| TEXAS INSTRUMENTS INCORPORATED
| Standard Linear and Logic Group
| IBIS Model of SN74AUCH16374
| 16-Bit Edge-Triggered D-Type Flip-Flop with 3-State Outputs
| This file contains package information for the following:
|  TSSOP 48-pin (DGG) package as [Component] AUCH16374_DGG
|  TVSOP 48-pin (DGV) package as [Component] AUCH16374_DGV
| This device can be powered at the following Vccs:
|  2.5 volt Vcc
|  1.8 volt Vcc
|  1.5 volt Vcc
|  1.2 volt Vcc
|  0.8 volt Vcc
| This file provides unique models under the [Model Selector] for each Vcc.
| For operation at a specific Vcc, select the appropriate model after each
| [Model Selector] keyword.
[IBIS Ver]   3.2
[Comment char]  |_char
[File Name]   sn74auch16374.ibs
[File Rev]   1.1 | x_die
[Date]   June 26, 2003
[Source]   Data created from TI-SPICE simulations at TI-SLL.
[Notes]   The following is an IBIS list for the AUCH16374.
   Please contact sllibis@ti.com with questions and
   comments concerning SLL IBIS models.
   -End point warning due to AC and DC mismatch.
   -Non-monotonic data in ground-clamp due to bus-hold
   -The waveforms for the AUCH16374_OUT Power Clamp ,Pullup,
   and Pulldown are caused by the circuitry that helps reduce
   overshoot and undershoot in transmission lines (EMI).
   These waveforms are norimal for this particular design.
   -Power clamp data deleted as there is no power-clamp diode.
[Disclaimer] Property of Texas Instruments Incorporated.  Unauthorized
   reproduction and/or distribution is strictly prohibited.
   This product is protected under copyright law.
   Created  2003, (C) Copyright  2003, Texas Instruments
   Incorporated, All Rights Reserved
   UNLESS THERE IS A SIGNED, WRITTEN AGREEMENT TO THE
   CONTRARY, TEXAS INSTRUMENTS (TI) IS PROVIDING THE IBIS
   MODELS  AND WITHOUT ANY WARRANTY, EXPRESSED OR
   IMPLIED.  TI assumes no liability for:
   1) the accuracy of the IBIS models provided to your
   company;
   2) the proper functioning of these IBIS Models in your
   design or for any resulting applications; or
   3) infringement of patents, copyrights or intellectual
   property rights resulting from your use of these IBIS
   models.
   TI provides IBIS Models as a service to our customers.
   You and your company shall not distribute, sell or give
   these models to anyone else without prior written
   permission from TI.
   TI reserves the right to make changes to our products or
   to discontinue any semiconductor product or service
   without notice, and advises our customers to obtain the
   latest version of relevant information to verify, before
   placing orders, that the information being relied on is
   current.
   Please be aware that your receipt and use of the IBIS
   information provided shall serve as acceptance of these
   terms and conditions.  If you do not accept these terms,
   you should return or destroy the IBIS models and any
   other accompanying information immediately.
| Component AUCH16374_DGG 48-pin TSSOP
[Component]   AUCH16374_DGG
[Manufacturer]   Texas Instruments, Inc.
[Package]
|   typ   min   max
R_pkg   6.200e-02   5.000e-02   7.800e-02
L_pkg   3.527e-09   3.128e-09   4.255e-09
C_pkg   5.300e-13   4.170e-13   6.850e-13
[Pin]   signal_name   model_name   R_pin   L_pin   C_pin
1   1NOE   AUCH16374_OEIN   5.000e-02   4.250e-09   6.710e-13
2   1Q1   AUCH16374_OUT   5.700e-02   3.956e-09   6.740e-13
3   1Q2   AUCH16374_OUT   7.100e-02   3.922e-09   6.190e-13
4   GND   GND   7.800e-02   3.841e-09   6.180e-13
5   1Q3   AUCH16374_OUT   5.600e-02   3.535e-09   5.550e-13
6   1Q4   AUCH16374_OUT   5.800e-02   3.464e-09   5.030e-13
7   VCC   POWER   6.000e-02   3.362e-09   4.980e-13
8   1Q5   AUCH16374_OUT   6.100e-02   3.293e-09   4.620e-13
9   1Q6   AUCH16374_OUT   6.300e-02   3.240e-09   4.550e-13
10   GND   GND   6.300e-02   3.175e-09   4.420e-13
11   1Q7   AUCH16374_OUT   6.400e-02   3.153e-09   4.290e-13
12   1Q8   AUCH16374_OUT   6.500e-02   3.128e-09   4.180e-13
13   2Q1   AUCH16374_OUT   6.500e-02   3.128e-09   4.180e-13
14   2Q2   AUCH16374_OUT   6.400e-02   3.154e-09   4.290e-13
15   GND   GND   6.300e-02   3.174e-09   4.420e-13
16   2Q3   AUCH16374_OUT   6.300e-02   3.241e-09   4.550e-13
17   2Q4   AUCH16374_OUT   6.100e-02   3.293e-09   4.620e-13
18   VCC   POWER   6.000e-02   3.362e-09   4.970e-13
19   2Q5   AUCH16374_OUT   5.800e-02   3.464e-09   5.030e-13
20   2Q6   AUCH16374_OUT   5.600e-02   3.537e-09   5.600e-13
21   GND   GND   7.700e-02   3.839e-09   6.260e-13
22   2Q7   AUCH16374_OUT   7.100e-02   3.917e-09   6.270e-13
23   2Q8   AUCH16374_OUT   5.800e-02   3.955e-09   6.850e-13
24   2NOE   AUCH16374_OEIN   5.200e-02   4.255e-09   6.790e-13
25   2CLK   AUCH16374_CLKIN   5.100e-02   4.254e-09   6.760e-13
26   2D8   AUCH16374_IN   5.800e-02   3.957e-09   6.790e-13
27   2D7   AUCH16374_IN   7.100e-02   3.920e-09   6.210e-13
28   GND   GND   7.800e-02   3.843e-09   6.220e-13
29   2D6   AUCH16374_IN   5.600e-02   3.539e-09   5.600e-13
30   2D5   AUCH16374_IN   5.800e-02   3.466e-09   5.030e-13
31   VCC   POWER   6.000e-02   3.363e-09   4.970e-13
32   2D4   AUCH16374_IN   6.100e-02   3.294e-09   4.620e-13
33   2D3   AUCH16374_IN   6.300e-02   3.241e-09   4.540e-13
34   GND   GND   6.300e-02   3.175e-09   4.410e-13
35   2D2   AUCH16374_IN   6.400e-02   3.153e-09   4.290e-13
36   2D1   AUCH16374_IN   6.500e-02   3.129e-09   4.170e-13
37   1D8   AUCH16374_IN   6.500e-02   3.129e-09   4.170e-13
38   1D7   AUCH16374_IN   6.400e-02   3.152e-09   4.290e-13
39   GND   GND   6.400e-02   3.176e-09   4.410e-13
40   1D6   AUCH16374_IN   6.300e-02   3.241e-09   4.540e-13
41   1D5   AUCH16374_IN   6.100e-02   3.293e-09   4.620e-13
42   VCC   POWER   6.000e-02   3.363e-09   4.970e-13
43   1D4   AUCH16374_IN   5.800e-02   3.464e-09   5.030e-13
44   1D3   AUCH16374_IN   5.600e-02   3.534e-09   5.610e-13
45   GND   GND   7.800e-02   3.841e-09   6.260e-13
46   1D2   AUCH16374_IN   7.100e-02   3.920e-09   6.220e-13
47   1D1   AUCH16374_IN   5.700e-02   3.955e-09   6.770e-13
48   1CLK   AUCH16374_CLKIN   5.100e-02   4.252e-09   6.720e-13
| Component AUCH16374_DGV 48-pin TVSOP
[Component]   AUCH16374_DGV
[Manufacturer]   Texas Instruments, Inc.
[Package]
|   typ   min   max
R_pkg   7.000e-02   4.900e-02   8.500e-02
L_pkg   3.013e-09   2.743e-09   3.408e-09
C_pkg   3.710e-13   2.940e-13   5.110e-13
[Pin]   signal_name   model_name   R_pin   L_pin   C_pin
1   1NOE   AUCH16374_OEIN   4.900e-02   3.393e-09   4.970e-13
2   1Q1   AUCH16374_OUT   6.000e-02   3.250e-09   5.020e-13
3   1Q2   AUCH16374_OUT   7.700e-02   3.310e-09   4.510e-13
4   GND   GND   8.500e-02   3.299e-09   4.040e-13
5   1Q3   AUCH16374_OUT   8.300e-02   3.136e-09   3.600e-13
6   1Q4   AUCH16374_OUT   7.700e-02   3.019e-09   3.630e-13
7   VCC   POWER   6.500e-02   2.882e-09   3.490e-13
8   1Q5   AUCH16374_OUT   6.600e-02   2.829e-09   3.140e-13
9   1Q6   AUCH16374_OUT   6.700e-02   2.796e-09   3.140e-13
10   GND   GND   6.900e-02   2.754e-09   3.080e-13
11   1Q7   AUCH16374_OUT   7.000e-02   2.753e-09   3.010e-13
12   1Q8   AUCH16374_OUT   7.100e-02   2.745e-09   2.940e-13
13   2Q1   AUCH16374_OUT   7.000e-02   2.744e-09   2.940e-13
14   2Q2   AUCH16374_OUT   7.000e-02   2.754e-09   3.010e-13
15   GND   GND   6.900e-02   2.754e-09   3.080e-13
16   2Q3   AUCH16374_OUT   6.700e-02   2.796e-09   3.140e-13
17   2Q4   AUCH16374_OUT   6.600e-02   2.829e-09   3.140e-13
18   VCC   POWER   6.500e-02   2.883e-09   3.500e-13
19   2Q5   AUCH16374_OUT   7.500e-02   3.014e-09   3.630e-13
20   2Q6   AUCH16374_OUT   8.000e-02   3.128e-09   3.580e-13
21   GND   GND   8.400e-02   3.295e-09   4.030e-13
22   2Q7   AUCH16374_OUT   7.800e-02   3.311e-09   4.520e-13
23   2Q8   AUCH16374_OUT   6.200e-02   3.259e-09   5.010e-13
24   2NOE   AUCH16374_OEIN   5.200e-02   3.404e-09   4.960e-13
25   2CLK   AUCH16374_CLKIN   5.300e-02   3.397e-09   5.050e-13
26   2D8   AUCH16374_IN   6.200e-02   3.249e-09   5.110e-13
27   2D7   AUCH16374_IN   7.700e-02   3.308e-09   4.530e-13
28   GND   GND   8.200e-02   3.289e-09   4.030e-13
29   2D6   AUCH16374_IN   7.800e-02   3.121e-09   3.590e-13
30   2D5   AUCH16374_IN   7.400e-02   3.010e-09   3.630e-13
31   VCC   POWER   6.500e-02   2.883e-09   3.490e-13
32   2D4   AUCH16374_IN   6.700e-02   2.829e-09   3.140e-13
33   2D3   AUCH16374_IN   6.700e-02   2.795e-09   3.140e-13
34   GND   GND   6.900e-02   2.753e-09   3.070e-13
35   2D2   AUCH16374_IN   7.000e-02   2.753e-09   3.010e-13
36   2D1   AUCH16374_IN   7.000e-02   2.743e-09   2.940e-13
37   1D8   AUCH16374_IN   7.000e-02   2.743e-09   2.940e-13
38   1D7   AUCH16374_IN   7.000e-02   2.753e-09   3.010e-13
39   GND   GND   6.900e-02   2.754e-09   3.070e-13
40   1D6   AUCH16374_IN   6.800e-02   2.797e-09   3.140e-13
41   1D5   AUCH16374_IN   6.700e-02   2.830e-09   3.140e-13
42   VCC   POWER   6.400e-02   2.880e-09   3.490e-13
43   1D4   AUCH16374_IN   7.200e-02   3.004e-09   3.620e-13
44   1D3   AUCH16374_IN   7.800e-02   3.121e-09   3.590e-13
45   GND   GND   8.400e-02   3.296e-09   4.030e-13
46   1D2   AUCH16374_IN   7.700e-02   3.308e-09   4.510e-13
47   1D1   AUCH16374_IN   6.200e-02   3.258e-09   4.990e-13
48   1CLK   AUCH16374_CLKIN   5.300e-02   3.408e-09   4.940e-13
| Model AUCH16374_CLKIN
[Model Selector]   AUCH16374_CLKIN
AUCH16374_CLKIN_25   2.5 volt Vcc
AUCH16374_CLKIN_18   1.8 volt Vcc
AUCH16374_CLKIN_15   1.5 volt Vcc
AUCH16374_CLKIN_12   1.2 volt Vcc
AUCH16374_CLKIN_08   0.8 volt Vcc
| Model AUCH16374_IN
[Model Selector]   AUCH16374_IN
AUCH16374_IN_25   2.5 volt Vcc
AUCH16374_IN_18   1.8 volt Vcc
AUCH16374_IN_15   1.5 volt Vcc
AUCH16374_IN_12   1.2 volt Vcc
AUCH16374_IN_08   0.8 volt Vcc
| Model AUCH16374_OEIN
[Model Selector]   AUCH16374_OEIN
AUCH16374_OEIN_25   2.5 volt Vcc
AUCH16374_OEIN_18   1.8 volt Vcc
AUCH16374_OEIN_15   1.5 volt Vcc
AUCH16374_OEIN_12   1.2 volt Vcc
AUCH16374_OEIN_08   0.8 volt Vcc
| Model AUCH16374_OUT
[Model Selector]   AUCH16374_OUT
AUCH16374_OUT_25   2.5 volt Vcc
AUCH16374_OUT_18   1.8 volt Vcc
AUCH16374_OUT_15   1.5 volt Vcc
AUCH16374_OUT_12   1.2 volt Vcc
AUCH16374_OUT_08   0.8 volt Vcc
| Models and submodels in the file (20): AUCH16374_CLKIN_25 (Input), AUCH16374_CLKIN_18 (Input), AUCH16374_CLKIN_15 (Input), AUCH16374_CLKIN_12 (Input), AUCH16374_CLKIN_08 (Input), AUCH16374_IN_25 (Input), AUCH16374_IN_18 (Input), AUCH16374_IN_15 (Input), AUCH16374_IN_12 (Input), AUCH16374_IN_08 (Input), AUCH16374_OEIN_25 (Input), AUCH16374_OEIN_18 (Input), AUCH16374_OEIN_15 (Input), AUCH16374_OEIN_12 (Input), AUCH16374_OEIN_08 (Input), AUCH16374_OUT_25 (3-state), AUCH16374_OUT_18 (3-state), AUCH16374_OUT_15 (3-state), AUCH16374_OUT_12 (3-state), AUCH16374_OUT_08 (3-state)
